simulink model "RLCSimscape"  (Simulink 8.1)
settings: Solver=ode23t  StartTime=0.0  StopTime=100  RelTol=1e-3
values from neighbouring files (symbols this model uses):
  U = 5    [MotorDCParam.m]
undefined symbols (not defined in the file or in its folder): R
libraries: fl_lib x6, nesl_utility x3

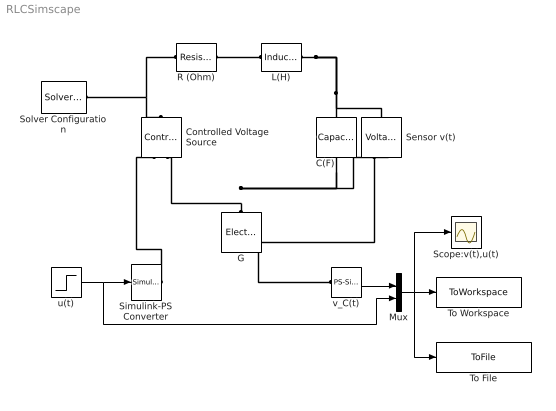
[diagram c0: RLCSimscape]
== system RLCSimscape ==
  C(F) : fl_lib/Electrical/Electrical Elements/Capacitor  c=C F  v0=0 V  r=0 Ohm  g=0 1/Ohm  i_Log=off  v_Log=off  vc_Log=off  LocalVarNames=|i|v|vc  LocalVarDescs=|i|v|Internal variable for voltage across capacitor term  LocalVarLogging=[0 0 0]
  Controlled Voltage Source : fl_lib/Electrical/Electrical Sources/Controlled Voltage Source  i_Log=off  v_Log=off  LocalVarNames=|i|v  LocalVarDescs=|i|v  LocalVarLogging=[0 0]
  G : fl_lib/Electrical/Electrical Elements/Electrical Reference  i_Log=off  LocalVarNames=|i  LocalVarDescs=|i  LocalVarLogging=0
  L(H) : fl_lib/Electrical/Electrical Elements/Inductor  l=L H  i0=0 A  r=0 Ohm  g=0 1/Ohm  i_Log=off  v_Log=off  i_L_Log=off  LocalVarNames=|i|v|i_L  LocalVarDescs=|i|v|Internal variable for current through inductor term  LocalVarLogging=[0 0 0]
  Mux : Mux  Inputs=2
  R (Ohm) : fl_lib/Electrical/Electrical Elements/Resistor  R=R Ohm  i_Log=off  v_Log=off  LocalVarNames=|i|v  LocalVarDescs=|i|v  LocalVarLogging=[0 0]
  Scope:v(t),u(t) : Scope
  Sensor v(t) : fl_lib/Electrical/Electrical Sensors/Voltage Sensor  i1_Log=off  v1_Log=off  LocalVarNames=|i1|v1  LocalVarDescs=|i1|v1  LocalVarLogging=[0 0]
  Simulink-PS Converter : nesl_utility/Simulink-PS Converter  PhysicalDomain=network_engine_domain  SubClassName=ps_input  LeftPortType=input  RightPortType=output  PseudoPeriodic=off  Frequencies=[]  NoiseDistribution=none  NoiseParameters=[]  Unit=V  AffineConversion=off  InputFiltering=off  SimscapeFilterOrder=1  InputFilterTimeConstant=0.001  UdotUserProvided=2
  Solver Configuration : nesl_utility/Solver Configuration  PhysicalDomain=network_engine_domain  SubClassName=solver  LeftPortType=input  RightPortType=generic  Accelerate=off  Tones=[]  Harmonics=[]  SimulateNoise=off  Profile=off  UseLocalSampling=off  EnableSwitchedLinearOptims=on  FrequencyDomain=off  UseCCode=off  UseNewInitialization=off  DoDC=off  ResidualTolerance=1e-09  UseLocalSolver=off  LocalSolverChoice=NE_TRAPEZOIDAL_ADVANCER  LocalSolverSampleTime=0.00001  DoFixedCost=on  MaxNonlinIter=3  MaxModeIter=2  LinearAlgebra=Sparse  DelaysMemoryBudget=1024
  To File : ToFile  Filename=RLCSimscape.mat  SaveFormat=Timeseries
  To Workspace : ToWorkspace  VariableName=RLCSimscape  SampleTime=-1
  u(t) : Step  Time=0  After=U  SampleTime=0
  v_C(t) : nesl_utility/PS-Simulink Converter  PhysicalDomain=network_engine_domain  SubClassName=ps_output  LeftPortType=input  RightPortType=output  PseudoPeriodic=off  Frequencies=[]  Unit=V  AffineConversion=off
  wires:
  Mux/1 -> To File/1, To Workspace/1, Scope:v(t),u(t)/1
  u(t)/1 -> Mux/2, Simulink-PS Converter/1
  v_C(t)/1 -> Mux/1
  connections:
  Solver Configuration/RConn1 -- R (Ohm)/LConn1 -- Controlled Voltage Source/LConn1
  L(H)/RConn1 -- Sensor v(t)/LConn1 -- C(F)/LConn1
  Simulink-PS Converter/RConn1 -- Controlled Voltage Source/RConn1
  Sensor v(t)/RConn1 -- v_C(t)/LConn1
  L(H)/LConn1 -- R (Ohm)/RConn1
  G/LConn1 -- Sensor v(t)/RConn2 -- C(F)/RConn1 -- Controlled Voltage Source/RConn2
